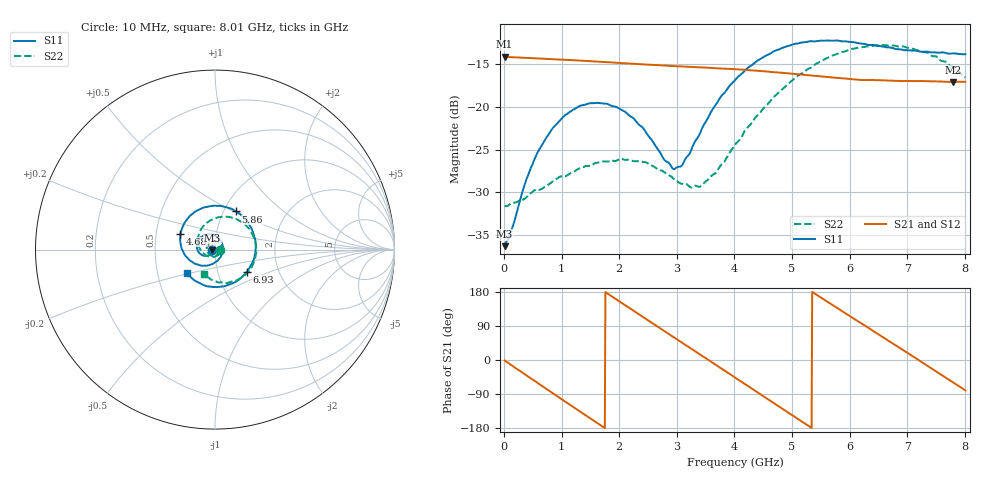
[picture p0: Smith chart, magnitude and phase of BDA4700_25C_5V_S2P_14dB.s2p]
!Agilent Technologies,E5071B,MY42404982,A.09.10
!Date: Mon Oct 20 13:33:11 2025
!Data & Calibration Information:
!Freq	S11:SOLT2(ON)	S21:SOLT2(ON)	S12:SOLT2(ON)	S22:SOLT2(ON)
# Hz S RI R 50
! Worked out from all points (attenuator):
!   801 points, 10 MHz to 8.01 GHz, reference 50 ohm
!   highest |S21| = -14.10 dB at 10 MHz (marker M1); lowest = -17.1 dB at 7.8 GHz (marker M2)
!   lowest |S11| = -36.3 dB at 10 MHz (marker M3), VSWR 1.03, Z = 48.5 - j0.132 ohm
!   |S11| at or under -10 dB: start of sweep to end of sweep
!   |S22| runs from -31.6 to -12.7 dB; largest |S21 - S12| = 0.0015
!   S11 on the Smith chart (normalised r, x): 10 MHz: 0.97, -0.00; 4.68 GHz: 0.67, +0.12; 5.86 GHz: 1.14, +0.51; 6.93 GHz: 1.38, -0.36; 8.01 GHz: 0.71, -0.19
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1e7  -0.0153 -0.00136  0.1972 -0.0043  0.1972 -0.00448  0.0264 -0.00104
1.5e8  -0.0169 -0.0106  0.1881 -0.0537  0.188 -0.0538  0.0262 -0.00768
3.9e8  -0.0269 -0.0267  0.1469 -0.1266  0.1468 -0.1268  0.0204 -0.0216
6e8  -0.043 -0.035  0.0892 -0.1705  0.0891 -0.1706  0.011 -0.0308
1e9  -0.0824 -0.0235  -0.0439 -0.1842  -0.0438 -0.1844  -0.0197 -0.034
1.35e9  -0.1015 0.013  -0.141 -0.1222  -0.1412 -0.1222  -0.0421 -0.013
1.71e9  -0.0869 0.0587  -0.1831 -0.0139  -0.1833 -0.0138  -0.0441 0.0189
2.07e9  -0.0431 0.0848  -0.153 0.096  -0.153 0.096  -0.0228 0.0438
2.68e9  0.0355 0.0435  0.00996 0.1755  0.00996 0.1754  0.0283 0.0323
2.93e9  0.0434 0.00279  0.0823 0.1531  0.0824 0.1529  0.0364 0.0122
3.08e9  0.0387 -0.0231  0.1186 0.1257  0.118 0.1261  0.0355 -0.00258
3.43e9  -0.00317 -0.0738  0.167 0.035  0.167 0.0349  0.0152 -0.031
4.01e9  -0.1251 -0.0704  0.1153 -0.1203  0.1154 -0.1201  -0.0505 -0.032
4.68e9  -0.1922 0.0887  -0.0636 -0.1467  -0.0634 -0.147  -0.0945 0.0641
5.35e9  -0.0545 0.2363  -0.1527 0.000508  -0.1528 6.74e-05  -0.00426 0.1714
5.86e9  0.1166 0.2125  -0.0941 0.1134  -0.0941 0.1135  0.1277 0.1664
6.25e9  0.2071 0.1099  -0.00569 0.1436  -0.00422 0.1438  0.2066 0.0883
6.68e9  0.2189 -0.0442  0.0913 0.1097  0.0916 0.1096  0.2263 -0.0331
6.93e9  0.1769 -0.1235  0.1274 0.0624  0.1276 0.0619  0.2018 -0.1024
7.36e9  0.0464 -0.2053  0.136 -0.0393  0.1361 -0.0395  0.1064 -0.178
7.8e9  -0.1052 -0.1775  0.0715 -0.1205  0.0714 -0.1209  -0.0155 -0.1696
8.01e9  -0.1578 -0.1292  0.0236 -0.1385  0.0238 -0.1386  -0.0593 -0.1363
